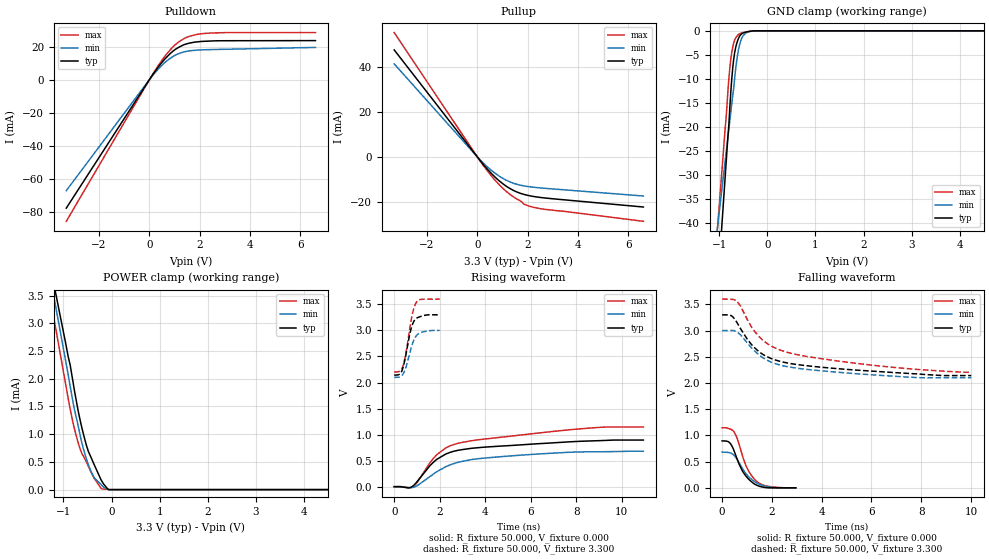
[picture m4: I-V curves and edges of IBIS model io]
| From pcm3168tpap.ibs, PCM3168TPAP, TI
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[Model]   io
Model_type I/O
Vinl=8.000E-01
Vinh=2.000E+00
Vref=0.000E+00
Rref=1.000E+06
Cref=0.000E+00
Vmeas=1.650E+00
C_comp   777.000fF   777.000fF   777.000fF
[Voltage Range]   3.300E+00   3.000E+00   3.600E+00
[POWER Clamp Reference]   3.300E+00   3.000E+00   3.600E+00
[GND Clamp Reference]   0.000E+00   0.000E+00   0.000E+00
[Pullup Reference]   3.300E+00   3.000E+00   3.600E+00
[Pulldown Reference]   0.000E+00   0.000E+00   0.000E+00
[Temperature Range]   25   105   -40
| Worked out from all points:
|   slope of the pulldown table from 0 to 0.495 V, typ, clamps not added: 47.9 ohm
|   slope of the pullup table from 0 to 0.495 V, typ, clamps not added: 75 ohm
|   GND clamp passes 1 mA (typ) near -0.57 V on its own axis
|   POWER clamp passes 1 mA (typ) near -0.58 V on its own axis
|   rising waveform, R_fixture 50.000, V_fixture 0.000: 20-80 % time 1.91ns typ, 2.48ns min, 2.79ns max; typ from 0 V to 0.895 V
|   falling waveform, R_fixture 50.000, V_fixture 0.000: 20-80 % time 570ps typ, 656ps min, 566ps max; typ from 0.895 V to 0 V
|   rising waveform, R_fixture 50.000, V_fixture 3.300: 20-80 % time 329ps typ, 362ps min, 321ps max; typ from 2.14 V to 3.3 V
|   falling waveform, R_fixture 50.000, V_fixture 3.300: 20-80 % time 2.02ns typ, 2.14ns min, 2.82ns max; typ from 3.3 V to 2.14 V
[GND Clamp]
-3.3V     -385.7mA   -236.3mA   -336.8mA
-880mV    -30.73mA   -27.26mA   -20.59mA
-800mV    -19.42mA   -20.35mA   -9.852mA
-780mV    -15.87mA   -18.62mA   -7.632mA
-740mV    -9.961mA   -15.16mA   -4.443mA
-720mV    -7.709mA   -13.43mA   -3.354mA
-660mV    -3.514mA   -7.992mA   -1.511mA
-620mV    -2.074mA   -5.051mA   -956.6uA
-560mV    -886.6uA   -2.284mA   -532.8uA
-440mV    -233.2uA   -396.9uA   -223.7uA
-280mV    0A         0A         0A
6.6V      0A         0A         0A
[Power Clamp]
-3.3V     12.83mA    13.4mA     13.34mA
-960mV    2.667mA    2.35mA     1.931mA
-900mV    2.393mA    2.064mA    1.638mA
-860mV    2.248mA    1.866mA    1.451mA
-760mV    1.731mA    1.402mA    1.057mA
-640mV    1.201mA    930.3uA    700.9uA
-580mV    984.6uA    720.8uA    594.8uA
-480mV    684.7uA    443.6uA    416.2uA
-360mV    448.8uA    211.8uA    202.8uA
-200mV    149.3uA    74.96uA    12.57uA
-60mV     0A         0A         0A
6.6V      0A         0A         0A
[Pullup]
-3.3V     47.49mA    41.29mA    55.2mA
180mV     -2.565mA   -2.087mA   -2.929mA
740mV     -9.368mA   -7.553mA   -10.81mA
1.06V     -12.33mA   -9.836mA   -14.46mA
1.3V      -14.1mA    -11.15mA   -16.68mA
1.74V     -16.33mA   -12.67mA   -19.79mA
1.84V     -16.66mA   -12.89mA   -20.9mA
2.34V     -17.8mA    -13.65mA   -22.68mA
6.6V      -22.3mA    -17.41mA   -28.65mA
[Pulldown]
-3.3V     -77.4mA    -66.86mA   -85.34mA
140mV     3.167mA    2.696mA    3.525mA
620mV     12.54mA    10.43mA    14.23mA
920mV     17.01mA    13.85mA    19.51mA
1.1V      18.97mA    15.3mA     22.02mA
1.5V      21.72mA    17.19mA    25.66mA
1.9V      22.83mA    17.86mA    27.34mA
2.2V      23.2mA     18.08mA    27.92mA
3.06V     23.53mA    18.38mA    28.44mA
6.6V      23.6mA     19.49mA    28.45mA
[Rising Waveform]
R_fixture = 50.000
V_fixture = 0.000
V_fixture_min = 0.000
V_fixture_max = 0.000
|  time   V(typ)   V(min)   V(max)
0s        0V         0V         0V
600ps     -22.83mV   -16.36mV   -17.51mV
840ps     19.05mV    -12.14mV   2.184mV
1.56ns    396.8mV    190.8mV    452mV
1.89ns    530.1mV    292.5mV    621.3mV
2.33ns    637.8mV    395.7mV    758.1mV
2.86ns    703.1mV    473.8mV    838.5mV
3.98ns    759mV      549.9mV    914.7mV
7.91ns    865.9mV    663.7mV    1.101V
10.95ns   895.1mV    681.1mV    1.146V
[Falling Waveform]
R_fixture = 50.000
V_fixture = 0.000
V_fixture_min = 0.000
V_fixture_max = 0.000
|  time   V(typ)   V(min)   V(max)
0s        895.1mV    681.1mV    1.146V
280ps     870.6mV    672.2mV    1.129V
500ps     681.2mV    609.5mV    1.052V
610ps     541mV      536.2mV    936mV
810ps     327.2mV    374.7mV    622.8mV
980ps     212.1mV    258.8mV    399.8mV
1.18ns    117.1mV    163.2mV    234.9mV
1.39ns    50.56mV    93.46mV    125mV
1.83ns    1.468mV    19.58mV    31.4mV
2.96ns    0V         0V         0V
[Rising Waveform]
R_fixture = 50.000
V_fixture = 3.300
V_fixture_min = 3.000
V_fixture_max = 3.600
|  time   V(typ)   V(min)   V(max)
0s        2.142V     2.099V     2.204V
250ps     2.164V     2.109V     2.22V
390ps     2.291V     2.164V     2.322V
520ps     2.545V     2.298V     2.576V
720ps     2.996V     2.623V     3.133V
790ps     3.102V     2.729V     3.298V
870ps     3.18V      2.823V     3.436V
970ps     3.23V      2.898V     3.537V
1.18ns    3.27V      2.96V      3.595V
2ns       3.3V       3V         3.6V
[Falling Waveform]
R_fixture = 50.000
V_fixture = 3.300
V_fixture_min = 3.000
V_fixture_max = 3.600
|  time   V(typ)   V(min)   V(max)
0s        3.3V       3V         3.6V
380ps     3.281V     3.002V     3.597V
580ps     3.167V     2.981V     3.568V
730ps     3.044V     2.923V     3.476V
1.02ns    2.828V     2.759V     3.202V
1.5ns     2.591V     2.529V     2.877V
1.95ns    2.471V     2.403V     2.712V
2.6ns     2.384V     2.313V     2.587V
6.22ns    2.221V     2.15V      2.33V
10.01ns   2.142V     2.099V     2.204V
[Ramp]
dV/dt_r   5.2957E-01/1.8780E-09   4.0232E-01/2.4679E-09   6.7583E-01/2.8000E-09
dV/dt_f   6.9475E-01/2.0178E-09   5.4036E-01/2.1344E-09   8.3763E-01/2.8124E-09
R_load = 50
